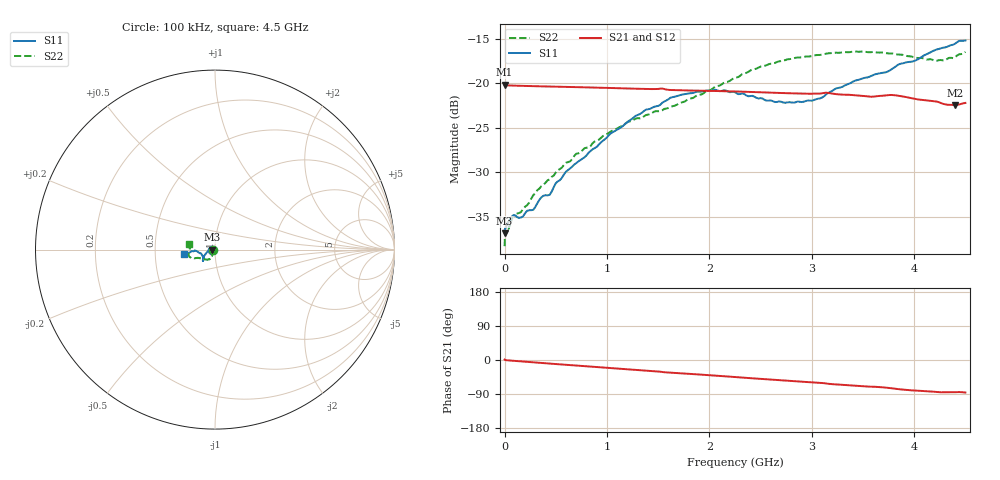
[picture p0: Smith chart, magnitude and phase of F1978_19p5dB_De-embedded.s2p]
! Integrated Device Technology
! Corporate Headquarters
! 6024 Silver Creek Valley Road
! San Jose, CA 95138  USA
! Phone:  1-408-284-8200
! Toll Free:  1-800-223-1366
! Webpage:  http://www.idt.com/
! Timing and RF Division
! 515 Groton Road, Suite 102
! Westford, MA 01886-6024
! Device:  F1978
! Description: 6-bit, 75 ohm, 0.5 dB Digital Step Attenuator
! Frequency:  5.0 MHz -  3.00 GHz
! Package:  4x4 mm QFN Plastic Package: 20 pin
! Ports:  2 RF, 11 DC
!  Pin  1  = D5 (16 dB)
!  Pin  2  = RF1  =  Port 1
!  Pin  3  = Serial Data In (DATA)
!  Pin  4  = Serial Clock (CLK)
!  Pin  5  = Serial Latch Enable (LE)
!  Pin  6  = VDD
!  Pin  7  = NC
!  Pin  8  = NC
!  Pin  9  = NC
!  Pin 10  = GND
!  Pin 11  = GND
!  Pin 12  = NC
!  Pin 13  = VMODE
!  Pin 14  = RF2  =  Port 2
!  Pin 15  = D4 (8 dB)
!  Pin 16  = D3 (4 dB)
!  Pin 17  = D2 (2 dB)
!  Pin 18  = NC
!  Pin 19  = D1 (1 dB)
!  Pin 20  = D0 (0.5 dB)
! State:  39
! Atten State:  19.5 dB
! Voltage:  +3.30 Volts
! Current:  0.564 mA
! Data:  The device was measured on a F1975 evaluation board which has
!  individual transmission lines to the RF pins.  Data was collected
!  using a calibrated network analyzer.  The evaluation board was
!  de-embedded using Automatic Fixture Removal (AFR).
!  The reference plane is the edge of the package pin.
! Misc:
!  Action Tracker AT0416
! Date Measured:  2018-02-08
! Date:  2018-03-26  MJV
! Note:
!  Integrated Device Technology supplies this data as a sample of measured
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# GHz S dB R 75
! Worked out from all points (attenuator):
!   291 points, 100 kHz to 4.5 GHz, reference 75 ohm
!   highest |S21| = -20.14 dB at 100 kHz (marker M1); lowest = -22.5 dB at 4.4 GHz (marker M2)
!   lowest |S11| = -36.9 dB at 100 kHz (marker M3), VSWR 1.03, Z = 72.9 - j0.00314 ohm
!   |S11| at or under -10 dB: start of sweep to end of sweep
!   |S22| runs from -38.3 to -16.4 dB; largest |S21 - S12| = 0.00019
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0.0001  -36.89 -179.9  -20.14 1.2  -20.14 1.2  -38.34 -178.6
0.003  -36.47 -178.0  -20.18 0.7  -20.18 0.7  -37.40 -176.0
0.01  -36.25 -178.4  -20.21 -0.4  -20.20 -0.4  -36.99 -173.6
0.1  -34.84 -174.8  -20.25 -2.4  -20.25 -2.4  -34.67 -153.9
0.16  -35.10 -176.5  -20.27 -3.7  -20.27 -3.7  -34.49 -144.0
0.28  -34.24 -179.3  -20.31 -6.2  -20.30 -6.2  -32.60 -133.4
0.36  -32.82 -179.2  -20.33 -7.8  -20.33 -7.8  -31.57 -125.9
0.44  -32.56 -178.2  -20.35 -9.4  -20.35 -9.4  -30.81 -120.6
0.6  -29.94 -174.7  -20.40 -12.7  -20.39 -12.7  -28.93 -117.7
0.76  -28.49 -167.6  -20.44 -15.9  -20.44 -15.9  -27.53 -116.6
1.28  -23.65 -151.7  -20.60 -26.2  -20.59 -26.2  -23.97 -120.1
1.52  -22.41 -143.9  -20.59 -30.9  -20.58 -30.9  -23.13 -127.3
1.62  -21.61 -142.3  -20.74 -33.2  -20.74 -33.2  -22.67 -130.9
1.88  -20.94 -138.3  -20.82 -37.9  -20.81 -37.9  -21.35 -142.6
2.26  -21.06 -137.8  -20.91 -45.1  -20.91 -45.2  -19.33 -154.1
2.64  -22.10 -147.2  -21.05 -52.4  -21.05 -52.4  -17.69 -158.4
3.02  -21.87 -163.8  -21.15 -59.3  -21.15 -59.2  -16.87 -162.0
3.42  -19.70 -175.1  -21.33 -67.9  -21.33 -67.9  -16.40 -168.5
3.76  -18.55 -175.7  -21.31 -74.0  -21.30 -74.0  -16.63 -175.6
4.2  -16.26 -172.7  -22.02 -83.9  -22.01 -83.9  -17.45 172.0
4.4  -15.52 -170.8  -22.45 -85.0  -22.45 -84.9  -17.05 168.7
4.5  -15.16 -172.6  -22.20 -85.9  -22.19 -85.8  -16.45 167.2
